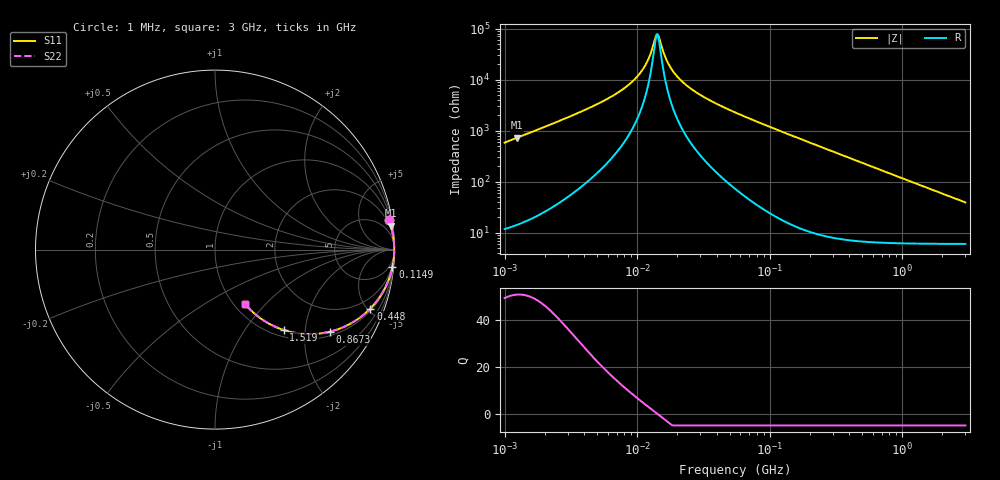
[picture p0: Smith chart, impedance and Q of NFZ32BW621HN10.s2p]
! NFZ32BW621HN10
# Hz S RI R 50
!Freq.(Hz) S11(Real) S11(Imag) S21(Real) S21(Imag) S12(Real) S12(Imag) S22(Real) S22(Imag)
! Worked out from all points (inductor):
!   401 points, 1 MHz to 3 GHz, reference 50 ohm
!   read as one part in series: L = 92.4 uH near 1.041 MHz
!   highest Q = 50.9 at 1.246 MHz (marker M1), where L = 93.2 uH
!   self-resonance near 14.04 MHz
!   S11 on the Smith chart (normalised r, x): 1 MHz: 1, +12; 114.9 MHz: 1, -21; 448 MHz: 1.14, -5.22; 867.3 MHz: 1.13, -2.69; 1.519 GHz: 1.12, -1.54; 3 GHz: 1.12, -0.78
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1000000  0.9684 0.1652  0.0316 -0.1652  0.0316 -0.1652  0.9684 0.1652
1246295  0.979 0.1338  0.021 -0.1338  0.021 -0.1338  0.979 0.1338
3823119  0.9968 0.0416  0.00315 -0.0416  0.00315 -0.0416  0.9968 0.0416
6563319  0.9983 0.0206  0.00174 -0.0206  0.00174 -0.0206  0.9983 0.0206
9223615  0.9986 0.0107  0.00141 -0.0107  0.00141 -0.0107  0.9986 0.0107
1.061086e7  0.9987 0.00713  0.00134 -0.00713  0.00134 -0.00713  0.9987 0.00713
1.172775e7  0.9987 0.00463  0.0013 -0.00463  0.0013 -0.00463  0.9987 0.00463
1.37644e7  0.9987 0.000727  0.00128 -0.000727  0.00128 -0.000727  0.9987 0.000727
1.404268e7  0.9987 0.000242  0.00128 -0.000242  0.00128 -0.000242  0.9987 0.000242
1.461624e7  0.9987 -0.000728  0.00128 0.000728  0.00128 0.000728  0.9987 -0.000728
1.615473e7  0.9987 -0.00316  0.00129 0.00316  0.00129 0.00316  0.9987 -0.00316
1.71545e7  0.9987 -0.00464  0.0013 0.00464  0.0013 0.00464  0.9987 -0.00464
2.137957e7  0.9986 -0.0102  0.00139 0.0102  0.00139 0.0102  0.9986 -0.0102
3.065274e7  0.9983 -0.0206  0.00173 0.0206  0.00173 0.0206  0.9983 -0.0206
5.477226e7  0.9967 -0.0435  0.0033 0.0435  0.0033 0.0435  0.9967 -0.0435
1.148668e8  0.9889 -0.0956  0.0111 0.0956  0.0111 0.0956  0.9889 -0.0956
2.094008e8  0.9662 -0.1719  0.0338 0.1719  0.0338 0.1719  0.9662 -0.1719
4.480278e8  0.8655 -0.3282  0.1345 0.3282  0.1345 0.3282  0.8655 -0.3282
8.005644e8  0.6738 -0.4477  0.3262 0.4477  0.3262 0.4477  0.6738 -0.4477
8.672962e8  0.6389 -0.4576  0.3611 0.4576  0.3611 0.4576  0.6389 -0.4576
1.519029e9  0.382 -0.4478  0.618 0.4478  0.618 0.4478  0.382 -0.4478
3e9  0.169 -0.305  0.831 0.305  0.831 0.305  0.169 -0.305
